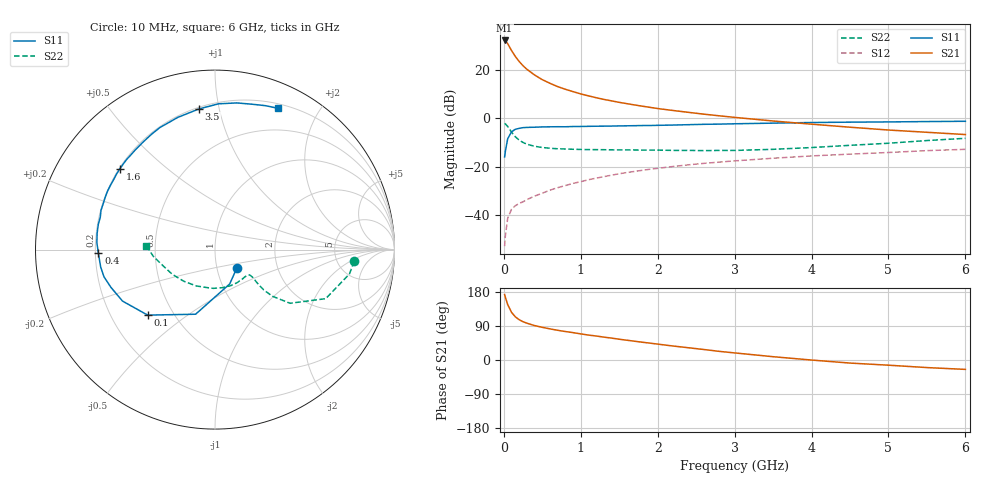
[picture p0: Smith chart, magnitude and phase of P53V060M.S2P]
! SIEMENS Small Signal Semiconductors
! BFP183
! Si NPN RF Bipolar Junction Transistor in SOT143
! VCE = 3 V  IC = 60 mA
! Common Emitter S-Parameters:  March  1996
# GHz  S  MA  R  50
!  f  S11  S21  S12  S22
! GHz  MAG  ANG  MAG  ANG  MAG  ANG  MAG  ANG
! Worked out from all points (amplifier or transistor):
!   36 points, 10 MHz to 6 GHz, reference 50 ohm
!   highest |S21| = 32.0 dB at 10 MHz (marker M1)
!   |S21| within 3 dB of that: start of sweep to 79.7 MHz
!   unconditionally stable (mu >= 1): start of sweep to 30.5 MHz; 212.2 MHz to end of sweep
!   at 250 MHz: K = 1.09, MAG = 26.2 dB, |S12| = -34.5 dB
!   at 1.4 GHz: K = 1.59, MAG = 10.8 dB, |S12| = -23.5 dB
!   at 6 GHz: K = 1.21, MAG = 0.3 dB, |S12| = -12.9 dB
!   S11 on the Smith chart (normalised r, x): 10 MHz: 1.25, -0.26; 100 MHz: 0.36, -0.36; 400 MHz: 0.21, -0.01; 1.6 GHz: 0.20, +0.35; 3.5 GHz: 0.21, +0.87; 6 GHz: 0.25, +1.51
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0.01  0.1586 -39.5  39.88 172.6  0.0023 67.3  0.7782 -4.8
0.02  0.2082 -66.8  39.17 165.5  0.0038 66.8  0.7611 -10.3
0.05  0.3759 -106.7  34.25 146.3  0.0086 64.7  0.6746 -23.9
0.1  0.5235 -135.8  24.74 125.7  0.0133 50.0  0.5138 -35.6
0.15  0.5898 -150.9  18.61 113.8  0.0157 48.2  0.412 -39.1
0.2  0.6169 -160.1  14.66 106.3  0.0175 49.9  0.352 -39.6
0.25  0.6367 -166.2  12 100.9  0.0189 49.8  0.3152 -38.9
0.3  0.6443 -171.3  10.14 97.1  0.021 52.0  0.2901 -37.9
0.4  0.6502 -178.3  7.746 90.8  0.0247 55.4  0.2629 -36.4
0.5  0.6593 176.6  6.2 86.2  0.0284 56.6  0.2482 -36.1
0.6  0.663 172.1  5.223 82.1  0.0328 59.4  0.2394 -36.3
0.7  0.6652 167.8  4.459 78.4  0.0369 60.6  0.2339 -37.1
0.9  0.6716 161.0  3.516 72.2  0.0453 61.4  0.2284 -39.9
1.1  0.6777 154.4  2.879 65.8  0.0538 61.8  0.2247 -43.5
1.3  0.6836 148.4  2.433 60.4  0.0623 60.9  0.2237 -48.1
1.6  0.6953 139.6  1.988 52.2  0.0757 59.3  0.2218 -55.2
2.2  0.7203 124.0  1.438 36.9  0.1008 54.1  0.2164 -72.4
2.8  0.7529 110.2  1.117 22.8  0.1241 48.0  0.2162 -92.3
3.5  0.7888 96.5  0.873 8.7  0.1493 41.1  0.2277 -117.2
4.5  0.8263 81.5  0.65 -8.1  0.1812 30.9  0.2753 -150.1
5.5  0.85 70.6  0.511 -20.0  0.214 21.7  0.3454 -173.7
6  0.8615 66.1  0.459 -24.8  0.2276 16.6  0.384 176.6
